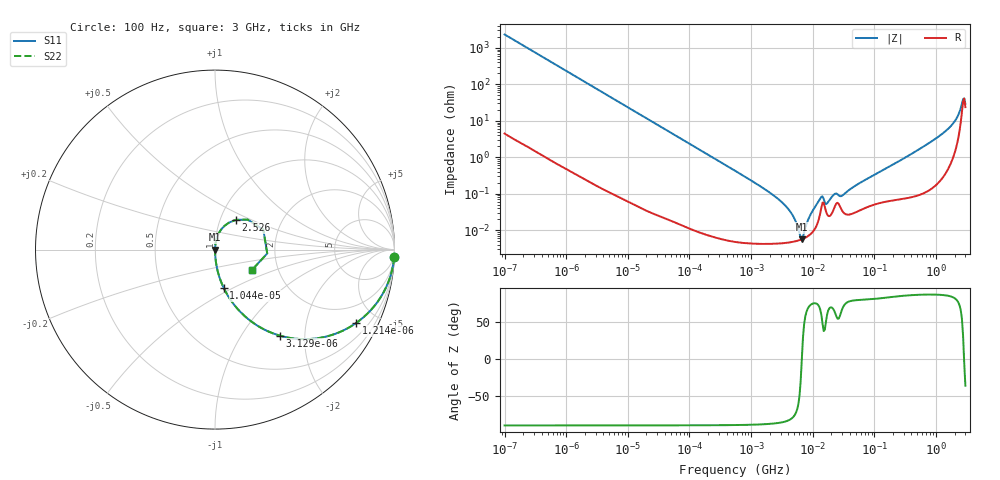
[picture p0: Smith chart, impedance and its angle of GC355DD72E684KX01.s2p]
!Murata Part Number: GC355DD72E684KX01
!These Parameters are Measured in Series Mode Connection
!Data Generated on Jan 08, 2026
!  o--ll--o
!Port1  Port2
!  o------o
!Operation Temp=25[degC], DC Bias Voltage=0[V]
!Freq. Start=100[Hz] Stop=3[GHz] 401[Steps]
# Hz S RI R 50
!Freq.(Hz) S11(Real) S11(Imag) S21(Real) S21(Imag) S12(Real) S12(Imag) S22(Real) S22(Imag)
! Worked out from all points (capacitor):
!   401 points, 100 Hz to 3 GHz, reference 50 ohm
!   read as one part in series: C = 682 nF near 109 Hz
!   lowest |Z| = 5.64 mohm at 6.649 MHz (marker M1)
!   series resonance near 2.852 GHz, so ESL is about 4.6 fH
!   S11 on the Smith chart (normalised r, x): 100 Hz: 1, -47; 1.214 kHz: 1.01, -3.86; 3.129 kHz: 1.00, -1.50; 10.44 kHz: 1.00, -0.45; 2.526 GHz: 1.18, +0.41; 3 GHz: 1.47, -0.35
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100  0.9981 -0.0428  0.00191 0.0428  0.00191 0.0428  0.9981 -0.0428
492  0.9573 -0.2012  0.0427 0.2012  0.0427 0.2012  0.9573 -0.2012
1214  0.7876 -0.408  0.2124 0.408  0.2124 0.408  0.7876 -0.408
1788  0.6315 -0.4813  0.3685 0.4813  0.3685 0.4813  0.6315 -0.4813
3129  0.3597 -0.4788  0.6403 0.4788  0.6403 0.4788  0.3597 -0.4788
10443  0.0486 -0.2138  0.9514 0.2138  0.9514 0.2138  0.0486 -0.2138
31977  0.00562 -0.0731  0.9944 0.0731  0.9944 0.0731  0.00562 -0.0731
547723  6.62e-05 -0.00429  0.9999 0.00429  0.9999 0.00429  6.62e-05 -0.00429
3063887  4.4e-05 -0.000613  1 0.000613  1 0.000613  4.4e-05 -0.000613
4323298  4.68e-05 -0.00032  1 0.00032  1 0.00032  4.68e-05 -0.00032
6648799  5.64e-05 0  0.9999 0  0.9999 0  5.64e-05 0
7565221  6.23e-05 9.7e-05  0.9999 -9.7e-05  0.9999 -9.7e-05  6.23e-05 9.7e-05
9794414  8.67e-05 0.000313  0.9999 -0.000313  0.9999 -0.000313  8.67e-05 0.000313
1.323817e7  0.000293 0.000685  0.9997 -0.000685  0.9997 -0.000685  0.000293 0.000685
1.713898e7  0.00027 0.000475  0.9997 -0.000475  0.9997 -0.000475  0.00027 0.000475
2.21892e7  0.000396 0.000873  0.9996 -0.000873  0.9996 -0.000873  0.000396 0.000873
2.999103e7  0.000343 0.000817  0.9997 -0.000817  0.9997 -0.000817  0.000343 0.000817
1.751444e8  0.000661 0.0055  0.9993 -0.0055  0.9993 -0.0055  0.000661 0.0055
1.324213e9  0.00513 0.0465  0.9949 -0.0465  0.9949 -0.0465  0.00513 0.0465
1.950712e9  0.0189 0.0869  0.9811 -0.0869  0.9811 -0.0869  0.0189 0.0869
2.525516e9  0.1152 0.1656  0.8848 -0.1656  0.8848 -0.1656  0.1152 0.1656
3e9  0.2075 -0.1116  0.7925 0.1116  0.7925 0.1116  0.2075 -0.1116
